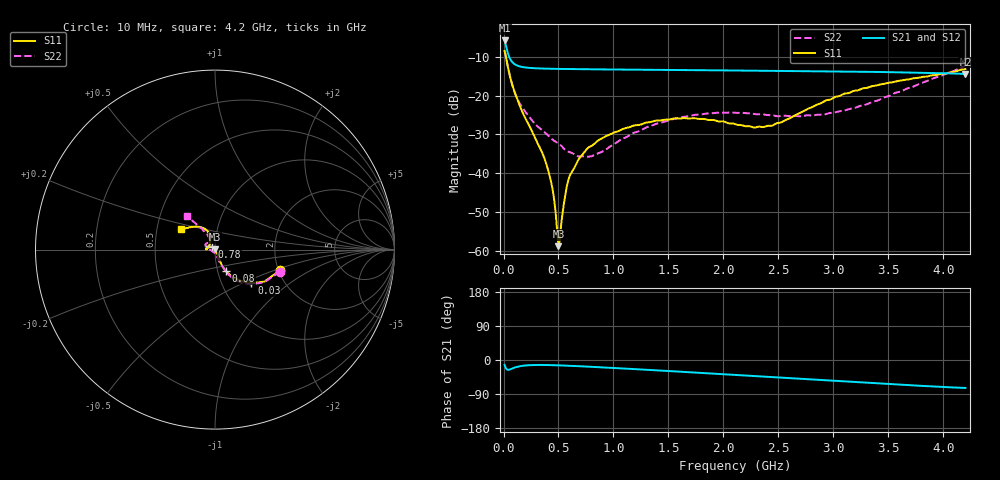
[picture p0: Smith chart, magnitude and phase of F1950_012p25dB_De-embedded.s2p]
! Integrated Device Technology
! Corporate Headquarters
! 6024 Silver Creek Valley Road
! San Jose, CA 95138  USA
! Phone:  1-408-284-8200
! Toll Free:  1-800-223-1366
! Webpage:  http://www.idt.com/
! Timing and RF Division
! 515 Groton Road, Suite 102
! Westford, MA 01886-6024
! Device:  F1950
! Description: 7-bit 0.25 dB Digital Step Attenuator
! Frequency:  150.0 -  4000.00 MHz
! Package:  4x4 mm Thin QFN Plastic Package: 24 pin
! Ports:  2 RF, 12 DC
!  Pin  1  = D0
!  Pin  2  = VDD
!  Pin  3  = Vmode
!  Pin  4  = GND
!  Pin  5  = RF1  =  Port 1
!  Pin  6  = GND
!  Pin  7  = GND
!  Pin  8  = GND
!  Pin  9  = GND
!  Pin 10  = GND
!  Pin 11  = GND
!  Pin 12  = GND
!  Pin 13  = GND
!  Pin 14  = RF2  =  Port 2
!  Pin 15  = GND
!  Pin 16  = LE
!  Pin 17  = CLK
!  Pin 18  = DATE
!  Pin 19  = D6
!  Pin 20  = D5
!  Pin 21  = D4
!  Pin 22  = D3
!  Pin 23  = D2
!  Pin 24  = D1
! State:  49
! Atten State:  12.25 dB
! Voltage:  +5.00 Volts
! Current:  Not Measured mA
! Data:  The device was measured on a the F195X evaluation board which has
!  individual transmission lines to the RF pins.  Data was collected
!  using a calibrated network analyzer.  The evaluation board was
!  de-embedded using a TRL calibration technique.
!  The reference plane is the edge of the package pin.
! Misc:  Board 2019
!  Action Tracker AT0250
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# GHz S dB R 50
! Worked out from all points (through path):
!   420 points, 10 MHz to 4.2 GHz, reference 50 ohm
!   highest |S21| = -5.74 dB at 10 MHz (marker M1); lowest = -14.4 dB at 4.2 GHz (marker M2)
!   group delay of S21, straight-line fit = 43.5 ps
!   lowest |S11| = -58.9 dB at 500 MHz (marker M3), VSWR 1.00, Z = 50.1 + j0.0676 ohm
!   |S11| at or under -10 dB: 22.2 MHz to end of sweep
!   |S22| runs from -35.8 to -8.4 dB; largest |S21 - S12| = 0.00031
!   S11 on the Smith chart (normalised r, x): 10 MHz: 2.03, -0.55; 30 MHz: 1.38, -0.56; 80 MHz: 1.10, -0.27; 780 MHz: 0.97, +0.03; 4.2 GHz: 0.66, +0.16
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0.01  -8.42 -17.8  -5.74 -12.9  -5.74 -12.9  -8.37 -18.8
0.03  -11.17 -42.8  -8.03 -24.7  -8.03 -24.7  -11.13 -44.2
0.08  -17.29 -62.6  -11.34 -22.4  -11.34 -22.4  -17.19 -63.5
0.18  -24.74 -65.3  -12.64 -15.1  -12.64 -15.1  -23.44 -70.9
0.39  -37.79 -52.5  -13.03 -13.2  -13.03 -13.3  -29.84 -76.9
0.44  -43.29 -46.7  -13.06 -13.6  -13.06 -13.6  -31.19 -80.2
0.49  -55.81 -1.2  -13.08 -14.0  -13.08 -14.0  -32.15 -85.9
0.5  -58.85 36.3  -13.09 -14.1  -13.09 -14.1  -32.32 -86.4
0.52  -54.41 100.5  -13.10 -14.3  -13.10 -14.3  -32.77 -87.3
0.56  -45.86 119.7  -13.11 -14.7  -13.11 -14.8  -33.98 -92.0
0.59  -41.74 126.7  -13.13 -15.1  -13.12 -15.1  -34.47 -98.3
0.71  -35.46 136.4  -13.16 -16.7  -13.16 -16.7  -35.67 -119.7
0.78  -33.23 139.7  -13.18 -17.7  -13.18 -17.7  -35.73 -134.2
1.09  -28.54 156.7  -13.27 -22.4  -13.27 -22.4  -31.04 -178.1
1.41  -26.42 170.5  -13.35 -27.6  -13.34 -27.6  -27.08 167.2
1.73  -25.81 177.7  -13.42 -32.9  -13.41 -33.0  -24.99 158.5
2.11  -27.39 170.3  -13.50 -39.5  -13.50 -39.5  -24.42 148.8
2.44  -27.76 135.9  -13.57 -45.1  -13.57 -45.1  -25.04 138.1
2.81  -22.91 111.1  -13.67 -51.6  -13.66 -51.6  -25.13 122.6
3.19  -18.73 113.3  -13.79 -58.3  -13.78 -58.3  -23.19 116.4
3.51  -16.63 122.0  -13.91 -63.6  -13.91 -63.7  -20.06 118.4
4.2  -13.09 149.4  -14.38 -73.7  -14.38 -73.8  -12.27 130.2
